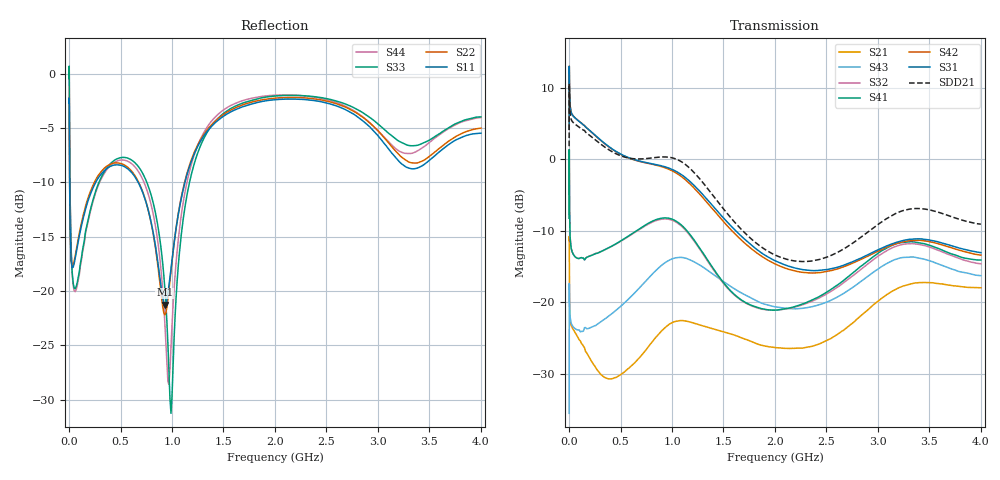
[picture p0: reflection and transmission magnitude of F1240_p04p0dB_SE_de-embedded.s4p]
! Integrated Device Technology
! Corporate Headquarters
! 6024 Silver Creek Valley Road
! San Jose, CA 95138  USA
! Phone:  1-408-284-8200
! Toll Free:  1-800-223-1366
! Webpage:  http://www.idt.com/
! Timing and RF Division
! 515 Groton Road, Suite 102
! Westford, MA 01886-6024
! Device:  F1240
! Description: Dual Intermediate Frequency Digital Variable Gain Amplifier
! Frequency:  10.0 -  500.00 MHz
! Package:  5x5 mm QFN Plastic Package: 32 pin
! Ports:  8 RF, 20 DC
!  Pin  1  = GA3 / Data  Pin 17  = RF OUT_B+
!  Pin  2  = GA4 / CLK  Pin 18  = RF OUT_B-
!  Pin  3  = GA5  Pin 19  = STBY_B
!  Pin  4  = VMODE  Pin 20  = Ground
!  Pin  5  = No Connect  Pin 21  = Ground
!  Pin  6  = GB5  Pin 22  = STB_A
!  Pin  7  = GB4  Pin 23  = RF OUT_A-  = Port 4
!  Pin  8  = GB3  Pin 24  = RF OUT_A+  = Port 3
!  Pin  9  = GB2  Pin 25  = GA0
!  Pin 10  = GB1  Pin 26  = ISET_A
!  Pin 11  = RF IN_B+  Pin 27  = VCC
!  Pin 12  = RF IN_B-  Pin 28  = Ground
!  Pin 13  = Ground  Pin 29  = RF IN_A-  = Port 2
!  Pin 14  = VCC  Pin 30  = RF IN_A+  = Port 1
!  Pin 15  = ISET_B  Pin 31  = GA1
!  Pin 16  = GB0  Pin 32  = GA2 / CSb
! Gain  = +19.5 dB
! State  = 1
! Voltage  = +5.00 V
! Current  = 85.292 mA (one channel only)
! Temperture  =  +25 C
! Test Date  =  2017-10-18
! Board  =  EB4031
! Data:  The device was measured on a custom evaluation board which has
!  individual transmission lines to the RF pins.  Data was collected
!  using a calibrated network analyzer.  The evaluation board was
!  de-embedded using Automatic Fixture Removal.
!  The reference plane is the edge of the package pin.
!  Only Channel A was measured.
!  This data is in single-ended operation.  If your needs are balanced
!  or differential S-parameters then this file needs to be used a
!  linear simulator.
! File Date:  2017-11-10  MJV
! Note:
!  Integrated Device Technology supplies this data as a sample of measured
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# Hz S dB R 100
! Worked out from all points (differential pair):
!   410 points, 500 kHz to 4 GHz, reference 100 ohm
!   strongest paths, dB at 500 kHz, 930 MHz, 1.96 GHz, 2.98 GHz, 4 GHz:
!     S31: 4.2, -1.0, -13.9, -12.8, -13.1
!     S42: 4.2, -1.2, -14.3, -13.0, -13.4
!     S41: -8.2, -8.2, -21.1, -13.4, -14.1
!     S32: -8.2, -8.3, -21.1, -13.8, -14.6
!     S43: -35.6, -14.5, -20.5, -15.6, -16.3
!     S21: -11.3, -23.6, -26.3, -20.1, -18.0
!   taken as a pair (ports 1,2 in; 3,4 out), SDD21 dB: 1.9, 0.4, -13.1, -9.3, -9.1
!   lowest |S11| = -21.3 dB at 930 MHz (marker M1), VSWR 1.19, Z = 85.2 - j6.14 ohm
!   |S11| at or under -10 dB: 5.625 MHz to 258.5 MHz (252.9 MHz wide, 191 % of centre); 671.3 MHz to 1.126 GHz (454.4 MHz wide, 50.6 % of centre)
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500000  -2.72 -5.5  -11.33 -5.8  -28.48 82.4  -42.38 79.3
        -11.34 -5.8  -2.71 -5.5  -42.40 78.4  -28.48 83.5
        4.23 -105.7  -8.24 -105.4  -0.44 1.2  -35.63 -60.6
        -8.23 -104.3  4.22 -104.5  -35.58 -60.4  -0.45 3.6
2500000  -4.30 -49.6  -14.47 -53.4  -17.36 31.1  -33.20 0.0
         -14.49 -53.4  -4.28 -49.6  -33.13 -0.4  -17.36 31.4
         12.63 -177.0  -0.20 161.7  -0.85 -51.3  -17.39 -148.8
         -0.24 161.7  12.62 -176.7  -17.36 -148.9  -0.91 -51.0
3e7  -17.88 -76.4  -23.55 -20.7  -17.62 -8.4  -39.92 -2.6
     -23.57 -20.9  -17.74 -77.3  -39.94 -2.5  -17.59 -8.4
     6.28 161.4  -12.93 144.0  -18.25 -127.5  -23.32 160.6
     -12.96 144.3  6.32 161.4  -23.25 160.7  -18.44 -128.0
1.8e8  -11.82 -123.1  -27.30 -49.5  -19.08 -46.9  -36.62 0.6
       -27.33 -49.0  -11.57 -124.3  -36.66 1.4  -19.10 -47.1
       4.32 114.0  -13.65 64.7  -13.66 -123.0  -23.81 104.0
       -13.66 64.9  4.32 113.4  -23.71 103.8  -13.79 -122.3
5.2e8  -8.48 -170.8  -30.21 -60.7  -20.49 -110.4  -31.32 -62.2
       -29.96 -59.6  -8.33 -172.4  -31.46 -60.1  -20.63 -110.9
       0.63 25.1  -11.31 -53.0  -7.70 -167.1  -20.63 11.9
       -11.26 -54.1  0.58 24.0  -20.34 11.8  -7.94 -167.4
9.3e8  -21.27 -155.6  -23.79 -109.2  -19.26 159.4  -28.61 -149.7
       -23.58 -112.7  -22.20 -154.9  -28.71 -143.4  -19.65 158.1
       -1.02 -77.6  -8.33 179.5  -19.74 143.7  -14.84 -90.6
       -8.19 176.3  -1.15 -79.8  -14.49 -91.2  -22.92 156.5
4e9  -5.48 -141.0  -18.01 100.4  -23.69 -56.8  -24.58 -38.8
     -17.98 100.1  -5.01 -139.7  -25.38 -22.5  -25.36 -50.8
     -13.05 28.7  -14.62 -80.4  -3.97 -136.3  -17.50 70.2
     -14.08 -94.2  -13.41 34.6  -16.29 58.4  -4.04 -145.5
